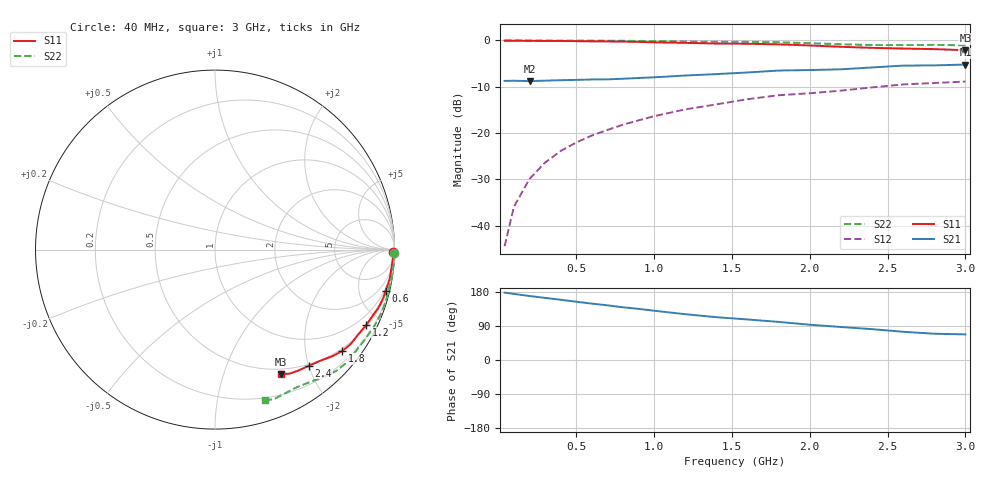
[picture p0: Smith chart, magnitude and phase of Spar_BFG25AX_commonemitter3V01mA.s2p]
! Filename:  BFG25AXF.S2P  Version:  2.0
! NXP part #: BFG25A/X  Date: May 1990
! Bias condition: Vce=3V, Ic=0.1mA
#  MHz  S  MA  R  50
! Freq  S11  S21  S12  S22  !GUM [dB]
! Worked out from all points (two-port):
!   21 points, 40 MHz to 3 GHz, reference 50 ohm
!   highest |S21| = -5.21 dB at 3 GHz (marker M1); lowest = -8.8 dB at 200 MHz (marker M2)
!   |S21| within 3 dB of the highest: 838.2 MHz to end of sweep
!   lowest |S11| = -2.1 dB at 3 GHz (marker M3), VSWR 8.26, Z = 21.9 - j78.8 ohm
!   |S11| at or under -10 dB: nowhere
!   |S22| runs from -1.1 to 0.0 dB; largest |S21 - S12| = 0.37
!   S11 on the Smith chart (normalised r, x): 40 MHz: open; 600 MHz: 0.79, -8.31; 1.2 GHz: 0.56, -4.19; 1.8 GHz: 0.44, -2.80; 2.4 GHz: 0.48, -2.00; 3 GHz: 0.44, -1.58
40  0.994 -0.9  0.366 177.9  0.006 89.2  1 -1.1
100  0.993 -2.3  0.367 174.3  0.016 87.7  1 -2.7
200  0.99 -4.6  0.364 168.9  0.032 85.7  0.998 -5.4
300  0.988 -6.8  0.368 163.9  0.048 83.6  0.996 -8.2
400  0.987 -9.1  0.372 159.0  0.064 82.0  0.995 -10.9
500  0.983 -11.3  0.375 153.8  0.079 80.2  0.995 -13.6
600  0.978 -13.6  0.379 148.8  0.094 78.7  0.994 -16.1
700  0.976 -15.7  0.38 144.3  0.108 77.2  0.993 -18.7
800  0.971 -17.9  0.386 139.1  0.123 75.6  0.991 -21.2
900  0.965 -19.9  0.393 135.0  0.137 74.0  0.988 -23.6
1000  0.955 -22.1  0.4 130.0  0.152 72.1  0.984 -26.1
1200  0.942 -26.4  0.418 120.9  0.18 67.7  0.973 -31.1
1400  0.927 -30.8  0.433 113.0  0.204 64.4  0.967 -36.1
1600  0.921 -35.0  0.451 107.0  0.232 62.0  0.966 -40.9
1800  0.907 -38.5  0.473 100.5  0.256 58.3  0.955 -45.1
2000  0.883 -42.3  0.479 93.1  0.269 54.5  0.935 -49.1
2200  0.854 -46.4  0.488 87.1  0.287 51.6  0.91 -53.8
2400  0.832 -51.0  0.511 81.4  0.311 47.2  0.892 -59.4
2600  0.818 -55.6  0.535 74.5  0.335 42.9  0.891 -64.5
2800  0.806 -59.1  0.538 69.3  0.347 40.4  0.896 -68.4
3000  0.784 -62.0  0.549 67.6  0.36 40.4  0.885 -71.6
